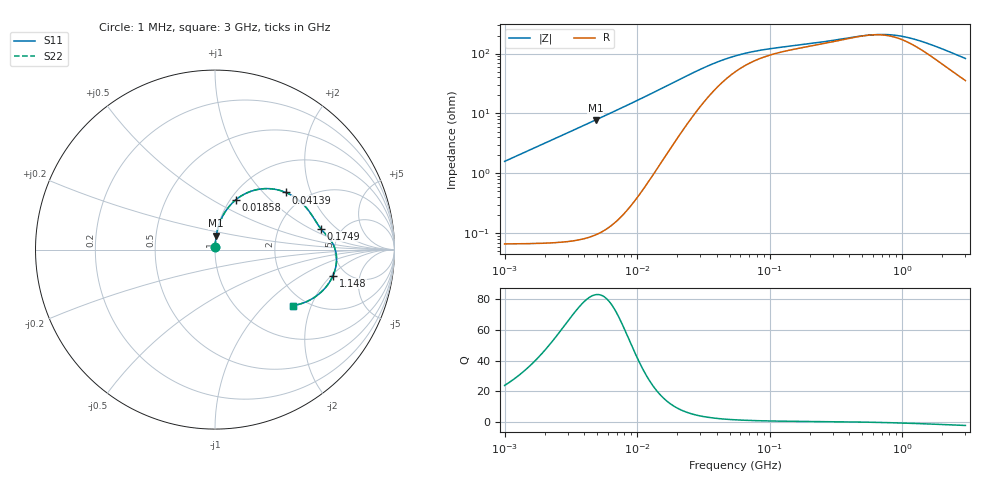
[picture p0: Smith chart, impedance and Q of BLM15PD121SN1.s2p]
! BLM15PD121SN1
# Hz S RI R 50
!Freq.(Hz) S11(Real) S11(Imag) S21(Real) S21(Imag) S12(Real) S12(Imag) S22(Real) S22(Imag)
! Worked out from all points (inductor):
!   401 points, 1 MHz to 3 GHz, reference 50 ohm
!   read as one part in series: L = 252 nH near 1.041 MHz
!   highest Q = 82.5 at 4.861 MHz (marker M1), where L = 255 nH
!   self-resonance near 558.9 MHz
!   S11 on the Smith chart (normalised r, x): 1 MHz: 1.00, +0.03; 18.58 MHz: 1.06, +0.65; 41.39 MHz: 1.58, +1.36; 174.9 MHz: 3.50, +1.28; 1.148 GHz: 3.96, -2.09; 3 GHz: 1.71, -1.49
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1000000  0.000916 0.0158  0.9991 -0.0158  0.9991 -0.0158  0.000916 0.0158
2097170  0.00179 0.0332  0.9982 -0.0332  0.9982 -0.0332  0.00179 0.0332
3823119  0.00449 0.0606  0.9955 -0.0606  0.9955 -0.0606  0.00449 0.0606
4861065  0.00694 0.0772  0.9931 -0.0772  0.9931 -0.0772  0.00694 0.0772
8686058  0.0222 0.1383  0.9778 -0.1383  0.9778 -0.1383  0.0222 0.1383
1.461624e7  0.069 0.2281  0.931 -0.2281  0.931 -0.2281  0.069 0.2281
1.858443e7  0.116 0.2774  0.884 -0.2774  0.884 -0.2774  0.116 0.2774
2.362996e7  0.1864 0.3197  0.8136 -0.3197  0.8136 -0.3197  0.1864 0.3197
2.829425e7  0.2524 0.3374  0.7476 -0.3374  0.7476 -0.3374  0.2524 0.3374
3.387922e7  0.3221 0.3377  0.6779 -0.3377  0.6779 -0.3377  0.3221 0.3377
4.138676e7  0.3935 0.3187  0.6065 -0.3187  0.6065 -0.3187  0.3935 0.3187
5.477226e7  0.4697 0.2721  0.5303 -0.2721  0.5303 -0.2721  0.4697 0.2721
8.507507e7  0.5368 0.1961  0.4632 -0.1961  0.4632 -0.1961  0.5368 0.1961
1.748812e8  0.5891 0.1171  0.4109 -0.1171  0.4109 -0.1171  0.5891 0.1171
2.094008e8  0.6009 0.1033  0.3991 -0.1033  0.3991 -0.1033  0.6009 0.1033
3.594878e8  0.6407 0.0578  0.3593 -0.0578  0.3593 -0.0578  0.6407 0.0578
5.364635e8  0.6677 0.00646  0.3323 -0.00646  0.3323 -0.00646  0.6677 0.00646
8.005644e8  0.6769 -0.0659  0.3231 0.0659  0.3231 0.0659  0.6769 -0.0659
1.147801e9  0.6577 -0.1445  0.3423 0.1445  0.3423 0.1445  0.6577 -0.1445
1.782824e9  0.5861 -0.2416  0.4139 0.2416  0.4139 0.2416  0.5861 -0.2416
2.359433e9  0.5112 -0.2894  0.4888 0.2894  0.4888 0.2894  0.5112 -0.2894
3e9  0.434 -0.3123  0.566 0.3123  0.566 0.3123  0.434 -0.3123
